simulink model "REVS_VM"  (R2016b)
settings: Solver=ode3  StartTime=REVS.sim_start_time_secs  StopTime=Inf  FixedStep=REVS.sim_step_time_secs  MaxStep=REVS.sim_step_time_secs  EnableMultiTasking=on
StopFcn:
  | postproc_datalog;
  | postproc_audit;
  | postproc_result;
model workspace (MATLAB code in the model file):
  other statements: REVS_setup_variants
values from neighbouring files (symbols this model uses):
  accessory = class_accessory_data    [class_test_data.m]
  battery = class_battery_data    [class_accessory_data.m]    (also in class_REVS_electric.m = class_REVS_battery)
  brake = struct(	'max_torque_Nm',[], 						'proportion_norm',1.0, 						'inertia_kgm2',0.0)    [class_REVS_drive_axle.m]
  engine = class_engine_data    [class_test_data.m]
  final_drive = struct(	'gear_ratio',[], 								'efficiency_norm',[], 								'inertia_kgm2',[] )    [class_REVS_drive_axle.m]
  gear = class_REVS_gearbox    [class_REVS_AT_transmission.m]
  tire = struct(	'radius_m',[], 						'rolling_resistance_coefficient',0, 						'vehicle_weight_norm',1.0,  						'wheel_slip_torque_Nm',[],  						'inertia_kgm2',0.0)    [class_REVS_drive_axle.m]
  torque_converter = class_REVS_torque_converter    [class_REVS_AT_transmission.m]
  transmission = class_transmission_data    [class_test_data.m]
  vehicle = class_vehicle_data    [class_test_data.m]
undefined symbols (not defined in the file or in its folder): alternator, ambient, controls, convert, DelayTimeSecs, drive_cycle, driver, electric, gear_strategy, InitialCondition, InitialValue, LoadSource, LookupStructure, MultiplyPosInputs, Normalize, NumPhases, REVS, SpeedSource, starter, tableshift, UpperSaturationLimit, Value, VerboseLevel, VerboseSignal
libraries: simulink x153
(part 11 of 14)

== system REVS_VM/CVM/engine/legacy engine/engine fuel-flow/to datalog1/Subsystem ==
  In1 : Inport
  Enable : EnablePort
  To Workspace : ToWorkspace  VariableName=datalog__engine__tipin_penalty_gps  SampleTime=-1
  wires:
  In1/1 -> To Workspace/1

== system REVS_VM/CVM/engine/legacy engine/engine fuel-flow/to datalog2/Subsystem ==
  In1 : Inport
  Enable : EnablePort
  To Workspace : ToWorkspace  VariableName=datalog__engine__base_fuel_rate_gps  SampleTime=-1
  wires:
  In1/1 -> To Workspace/1

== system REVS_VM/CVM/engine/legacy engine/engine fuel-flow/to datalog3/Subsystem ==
  In1 : Inport
  Enable : EnablePort
  To Workspace : ToWorkspace  VariableName=datalog__engine__twoD_eng_trq_Nm  SampleTime=-1
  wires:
  In1/1 -> To Workspace/1

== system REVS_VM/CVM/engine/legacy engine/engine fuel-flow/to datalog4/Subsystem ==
  In1 : Inport
  Enable : EnablePort
  To Workspace : ToWorkspace  VariableName=datalog__engine__twoD_eng_spd_radps  SampleTime=-1
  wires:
  In1/1 -> To Workspace/1

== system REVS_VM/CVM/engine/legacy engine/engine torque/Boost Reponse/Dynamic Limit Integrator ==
  upper : Inport
  In : Inport  Port=2
  rst : Inport  Port=3
  Xo : Inport  Port=4
  lower : Inport  Port=5
  Integrator : Integrator  ExternalReset=level  InitialConditionSource=external  ShowStatePort=on
  Logical Operator : Logic  Operator=OR  Inputs=3  AllPortsSameDT=off  OutDataTypeStr=boolean
  lower limit : MinMax  Function=max  Inputs=2  ZeroCross=off
  lower saturation : RelationalOperator  Operator=<  OutDataTypeStr=boolean
  manual reset : Switch  Criteria=u2 ~= 0
  upper limit : MinMax  Inputs=2
  upper saturation : RelationalOperator  Operator=>  OutDataTypeStr=boolean
  Out : Outport
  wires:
  manual reset/1 -> lower limit/1
  upper/1 -> upper limit/1, upper saturation/2
  upper limit/1 -> Integrator/3
  lower/1 -> lower saturation/2, lower limit/2
  In/1 -> Integrator/1
  Logical Operator/1 -> Integrator/2
  lower saturation/1 -> Logical Operator/2
  upper saturation/1 -> Logical Operator/1
  rst/1 -> Logical Operator/3, manual reset/2
  Xo/1 -> manual reset/1
  lower limit/1 -> upper limit/2
  Integrator/1 -> Out/1
  Integrator/State -> upper saturation/1, lower saturation/1, manual reset/3

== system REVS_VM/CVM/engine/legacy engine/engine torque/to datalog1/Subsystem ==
  In1 : Inport
  Enable : EnablePort
  To Workspace : ToWorkspace  VariableName=datalog__engine__load_Nm  SampleTime=-1
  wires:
  In1/1 -> To Workspace/1

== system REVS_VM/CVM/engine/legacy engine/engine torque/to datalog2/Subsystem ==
  In1 : Inport
  Enable : EnablePort
  To Workspace : ToWorkspace  VariableName=datalog__engine__load_norm  SampleTime=-1
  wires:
  In1/1 -> To Workspace/1

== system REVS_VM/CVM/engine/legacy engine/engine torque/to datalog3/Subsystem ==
  In1 : Inport
  Enable : EnablePort
  To Workspace : ToWorkspace  VariableName=datalog__engine__available_torque_Nm  SampleTime=-1
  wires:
  In1/1 -> To Workspace/1

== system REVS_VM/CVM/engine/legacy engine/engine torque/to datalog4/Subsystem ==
  In1 : Inport
  Enable : EnablePort
  To Workspace : ToWorkspace  VariableName=datalog__engine__fueling_torque_Nm  SampleTime=-1
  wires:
  In1/1 -> To Workspace/1

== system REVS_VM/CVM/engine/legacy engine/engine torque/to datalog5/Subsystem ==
  In1 : Inport
  Enable : EnablePort
  To Workspace : ToWorkspace  VariableName=datalog__engine__slow_target_torque_Nm  SampleTime=-1
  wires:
  In1/1 -> To Workspace/1

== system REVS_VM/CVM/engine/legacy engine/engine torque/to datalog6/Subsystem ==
  In1 : Inport
  Enable : EnablePort
  To Workspace : ToWorkspace  VariableName=datalog__engine__fast_target_torque_Nm  SampleTime=-1
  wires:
  In1/1 -> To Workspace/1

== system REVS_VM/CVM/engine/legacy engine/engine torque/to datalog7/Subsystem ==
  In1 : Inport
  Enable : EnablePort
  To Workspace : ToWorkspace  VariableName=datalog__engine__naturally_aspirated_torque_Nm  SampleTime=-1
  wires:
  In1/1 -> To Workspace/1

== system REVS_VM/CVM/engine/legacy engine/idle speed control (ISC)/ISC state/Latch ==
  On : Inport  PortDimensions=1
  Off : Inport  Port=2  PortDimensions=1
  Combinatorial  Logic : CombinatorialLogic  TruthTable=[0;1;0;0;1;1;(tb==2);(tb>=2)]
  Memory2 : Memory  X0=InitialCondition
  Mux : Mux  Inputs=3
  State : Outport  PortDimensions=1
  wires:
  Off/1 -> Mux/2
  On/1 -> Mux/1
  Memory2/1 -> Mux/3
  Mux/1 -> Combinatorial  Logic/1
  Combinatorial  Logic/1 -> State/1, Memory2/1

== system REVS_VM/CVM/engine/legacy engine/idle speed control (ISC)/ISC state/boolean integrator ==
  bool : Inport
  Constant : Constant  Value=Normalize
  Data Type Conversion2 : DataTypeConversion  OutDataTypeStr=double
  Integrator1 : Integrator  ExternalReset=falling  LimitOutput=on  UpperSaturationLimit=UpperSaturationLimit  LowerSaturationLimit=0
  Switch : Switch  Criteria=u2 > Threshold
  normalize : Gain  Gain=1/UpperSaturationLimit
  out : Outport
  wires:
  Switch/1 -> out/1
  normalize/1 -> Switch/1
  Integrator1/1 -> Switch/3, normalize/1
  Constant/1 -> Switch/2
  bool/1 -> Data Type Conversion2/1
  Data Type Conversion2/1 -> Integrator1/1, Integrator1/2

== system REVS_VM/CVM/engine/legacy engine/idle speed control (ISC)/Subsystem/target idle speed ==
  bus : Inport
  Bus Selector : BusSelector  OutputSignals=gb.gb_cmd_gear,gb_spd_in_radps,ctrl.gb_line_press_bar
  Lookup : Lookup_n-D  NumberOfTableDimensions=10  BreakpointsForDimension1=LookupStructure.axis_1.breakpoints  BreakpointsForDimension2=LookupStructure.axis_2.breakpoints  BreakpointsForDimension3=LookupStructure.axis_3.breakpoints  BreakpointsForDimension4=LookupStructure.axis_4.breakpoints  BreakpointsForDimension5=LookupStructure.axis_5.breakpoints  BreakpointsForDimension6=LookupStructure.axis_6.breakpoints  BreakpointsForDimension7=LookupStructure.axis_7.breakpoints  BreakpointsForDimension8=LookupStructure.axis_8.breakpoints  BreakpointsForDimension9=LookupStructure.axis_9.breakpoints  BreakpointsForDimension10=LookupStructure.axis_10.breakpoints  IndexSearchMethod=Linear search  BeginIndexSearchUsingPreviousIndexResult=on  Table=LookupStructure.table  InternalRulePriority=Speed  RndMeth=Simplest  SupportTunableTableSize=on  MaximumIndicesForEachDimension=LookupStructure.table_size
  out : Outport
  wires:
  bus/1 -> Bus Selector/1
  Lookup/1 -> out/1

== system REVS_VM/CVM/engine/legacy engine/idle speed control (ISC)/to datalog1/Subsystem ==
  In1 : Inport
  Enable : EnablePort
  To Workspace : ToWorkspace  VariableName=datalog__engine__ISC_torque_Nm  SampleTime=-1
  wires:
  In1/1 -> To Workspace/1

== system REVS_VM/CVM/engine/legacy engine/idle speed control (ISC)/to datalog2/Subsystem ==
  In1 : Inport
  Enable : EnablePort
  To Workspace : ToWorkspace  VariableName=datalog__engine__ISC_Ki_torque_Nm  SampleTime=-1
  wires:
  In1/1 -> To Workspace/1

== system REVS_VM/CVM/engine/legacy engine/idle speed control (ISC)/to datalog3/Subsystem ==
  In1 : Inport
  Enable : EnablePort
  To Workspace : ToWorkspace  VariableName=datalog__engine__ISC_Kp_torque_Nm  SampleTime=-1
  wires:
  In1/1 -> To Workspace/1

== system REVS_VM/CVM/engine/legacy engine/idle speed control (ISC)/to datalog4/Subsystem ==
  In1 : Inport
  Enable : EnablePort
  To Workspace : ToWorkspace  VariableName=datalog__engine__ISC_Ialpha_Nm  SampleTime=-1
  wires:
  In1/1 -> To Workspace/1

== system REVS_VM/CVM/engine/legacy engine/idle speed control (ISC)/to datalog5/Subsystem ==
  In1 : Inport
  Enable : EnablePort
  To Workspace : ToWorkspace  VariableName=datalog__engine__ISC_target_speed_radps  SampleTime=-1
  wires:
  In1/1 -> To Workspace/1

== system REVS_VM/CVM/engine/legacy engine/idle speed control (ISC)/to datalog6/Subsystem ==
  In1 : Inport
  Enable : EnablePort
  To Workspace : ToWorkspace  VariableName=datalog__engine__ISC_state  SampleTime=-1
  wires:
  In1/1 -> To Workspace/1

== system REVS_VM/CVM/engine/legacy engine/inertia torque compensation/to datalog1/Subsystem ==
  In1 : Inport
  Enable : EnablePort
  To Workspace : ToWorkspace  VariableName=datalog__engine__inertia_comp_torque_Nm  SampleTime=-1
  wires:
  In1/1 -> To Workspace/1

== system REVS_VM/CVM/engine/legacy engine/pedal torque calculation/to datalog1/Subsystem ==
  In1 : Inport
  Enable : EnablePort
  To Workspace : ToWorkspace  VariableName=datalog__engine__accel_pedal_torque_Nm  SampleTime=-1
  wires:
  In1/1 -> To Workspace/1

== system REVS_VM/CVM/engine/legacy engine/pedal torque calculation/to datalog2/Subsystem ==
  In1 : Inport
  Enable : EnablePort
  To Workspace : ToWorkspace  VariableName=datalog__engine__accel_pedal_power_W  SampleTime=-1
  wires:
  In1/1 -> To Workspace/1

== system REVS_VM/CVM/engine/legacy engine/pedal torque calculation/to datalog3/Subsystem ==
  In1 : Inport
  Enable : EnablePort
  To Workspace : ToWorkspace  VariableName=datalog__engine__current_available_power_W  SampleTime=-1
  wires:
  In1/1 -> To Workspace/1

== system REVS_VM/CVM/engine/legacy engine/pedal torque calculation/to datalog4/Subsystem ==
  In1 : Inport
  Enable : EnablePort
  To Workspace : ToWorkspace  VariableName=datalog__engine__current_available_torque_Nm  SampleTime=-1
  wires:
  In1/1 -> To Workspace/1

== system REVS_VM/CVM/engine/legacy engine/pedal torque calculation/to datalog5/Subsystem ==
  In1 : Inport
  Enable : EnablePort
  To Workspace : ToWorkspace  VariableName=datalog__engine__current_min_torque_Nm  SampleTime=-1
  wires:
  In1/1 -> To Workspace/1

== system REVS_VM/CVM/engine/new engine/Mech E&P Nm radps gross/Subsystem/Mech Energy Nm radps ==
  trq_Nm : Inport
  spd_radps : Inport  Port=2
  Gain : Gain  Gain=-1
  Integrator : Integrator  ZeroCross=off
  Integrator1 : Integrator  ZeroCross=off
  Integrator2 : Integrator  ZeroCross=off
  Mux : Mux  Inputs=2
  Neg : Fcn  Expr=u(1)*(u(1) <= 0)
  Pos : Fcn  Expr=u(1)*(u(1) >= 0)
  calc_Power_kW : Fcn  Expr=u(1)*u(2)/1000
  "total_kJ " : Outport
  "pos_kJ " : Outport  Port=2
  neg_kJ : Outport  Port=3
  pwr_kW : Outport  Port=4
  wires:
  calc_Power_kW/1 -> Pos/1, Neg/1, pwr_kW/1, Integrator/1
  Gain/1 -> neg_kJ/1
  Integrator1/1 -> "pos_kJ "/1
  Integrator2/1 -> Gain/1
  Neg/1 -> Integrator2/1
  Pos/1 -> Integrator1/1
  spd_radps/1 -> Mux/2
  trq_Nm/1 -> Mux/1
  Mux/1 -> calc_Power_kW/1
  Integrator/1 -> "total_kJ "/1

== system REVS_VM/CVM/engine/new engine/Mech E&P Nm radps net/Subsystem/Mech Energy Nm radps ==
  trq_Nm : Inport
  spd_radps : Inport  Port=2
  Gain : Gain  Gain=-1
  Integrator : Integrator  ZeroCross=off
  Integrator1 : Integrator  ZeroCross=off
  Integrator2 : Integrator  ZeroCross=off
  Mux : Mux  Inputs=2
  Neg : Fcn  Expr=u(1)*(u(1) <= 0)
  Pos : Fcn  Expr=u(1)*(u(1) >= 0)
  calc_Power_kW : Fcn  Expr=u(1)*u(2)/1000
  "total_kJ " : Outport
  "pos_kJ " : Outport  Port=2
  neg_kJ : Outport  Port=3
  pwr_kW : Outport  Port=4
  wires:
  calc_Power_kW/1 -> Pos/1, Neg/1, pwr_kW/1, Integrator/1
  Gain/1 -> neg_kJ/1
  Integrator1/1 -> "pos_kJ "/1
  Integrator2/1 -> Gain/1
  Neg/1 -> Integrator2/1
  Pos/1 -> Integrator1/1
  spd_radps/1 -> Mux/2
  trq_Nm/1 -> Mux/1
  Mux/1 -> calc_Power_kW/1
  Integrator/1 -> "total_kJ "/1

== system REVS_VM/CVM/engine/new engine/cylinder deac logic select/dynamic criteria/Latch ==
  On : Inport  PortDimensions=1
  Off : Inport  Port=2  PortDimensions=1
  Combinatorial  Logic : CombinatorialLogic  TruthTable=[0;1;0;0;1;1;(tb==2);(tb>=2)]
  Memory2 : Memory  X0=InitialCondition
  Mux : Mux  Inputs=3
  State : Outport  PortDimensions=1
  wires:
  Off/1 -> Mux/2
  On/1 -> Mux/1
  Memory2/1 -> Mux/3
  Mux/1 -> Combinatorial  Logic/1
  Combinatorial  Logic/1 -> State/1, Memory2/1

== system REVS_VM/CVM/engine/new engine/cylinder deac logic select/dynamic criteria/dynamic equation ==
  bus : Inport
  Bus Creator : BusCreator  Inputs=10
  Bus Creator1 : BusCreator  Inputs=2
  Bus Selector : BusSelector  OutputSignals=var_sigs.var_sig1  OutputAsBus=on
  Data Type Conversion : DataTypeConversion  OutDataTypeStr=double
  Display : Display
  Fcn : Fcn
  Variable {1..10} (10 alike) : Constant  Value=nan
  out : Outport
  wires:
  Data Type Conversion/1 -> Fcn/1
  Bus Selector/1 -> Data Type Conversion/1, Display/1
  Bus Creator1/1 -> Bus Selector/1
  Fcn/1 -> out/1
  bus/1 -> Bus Creator1/1  "system_bus"
  Bus Creator/1 -> Bus Creator1/2  "var_sigs"
  Variable 1/1 -> Bus Creator/1  "var_sig1"
  Variable 2/1 -> Bus Creator/2  "var_sig2"
  Variable 3/1 -> Bus Creator/3  "var_sig3"
  Variable 4/1 -> Bus Creator/4  "var_sig4"
  Variable 5/1 -> Bus Creator/5  "var_sig5"
  Variable 6/1 -> Bus Creator/6  "var_sig6"
  Variable 7/1 -> Bus Creator/7  "var_sig7"
  Variable 8/1 -> Bus Creator/8  "var_sig8"
  Variable 9/1 -> Bus Creator/9  "var_sig9"
  Variable 10/1 -> Bus Creator/10  "var_sig10"

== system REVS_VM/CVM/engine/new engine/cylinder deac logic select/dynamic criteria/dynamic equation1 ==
  bus : Inport
  Bus Creator : BusCreator  Inputs=10
  Bus Creator1 : BusCreator  Inputs=2
  Bus Selector : BusSelector  OutputSignals=var_sigs.var_sig1  OutputAsBus=on
  Data Type Conversion : DataTypeConversion  OutDataTypeStr=double
  Display : Display
  Fcn : Fcn
  Variable {1..10} (10 alike) : Constant  Value=nan
  out : Outport
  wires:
  Data Type Conversion/1 -> Fcn/1
  Bus Selector/1 -> Data Type Conversion/1, Display/1
  Bus Creator1/1 -> Bus Selector/1
  Fcn/1 -> out/1
  bus/1 -> Bus Creator1/1  "system_bus"
  Bus Creator/1 -> Bus Creator1/2  "var_sigs"
  Variable 1/1 -> Bus Creator/1  "var_sig1"
  Variable 2/1 -> Bus Creator/2  "var_sig2"
  Variable 3/1 -> Bus Creator/3  "var_sig3"
  Variable 4/1 -> Bus Creator/4  "var_sig4"
  Variable 5/1 -> Bus Creator/5  "var_sig5"
  Variable 6/1 -> Bus Creator/6  "var_sig6"
  Variable 7/1 -> Bus Creator/7  "var_sig7"
  Variable 8/1 -> Bus Creator/8  "var_sig8"
  Variable 9/1 -> Bus Creator/9  "var_sig9"
  Variable 10/1 -> Bus Creator/10  "var_sig10"

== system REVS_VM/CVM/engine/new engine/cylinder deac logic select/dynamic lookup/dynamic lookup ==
  bus : Inport
  Bus Selector : BusSelector  OutputSignals=gb.gb_cmd_gear,gb_spd_in_radps,ctrl.gb_line_press_bar
  Lookup : Lookup_n-D  NumberOfTableDimensions=10  BreakpointsForDimension1=LookupStructure.axis_1.breakpoints  BreakpointsForDimension2=LookupStructure.axis_2.breakpoints  BreakpointsForDimension3=LookupStructure.axis_3.breakpoints  BreakpointsForDimension4=LookupStructure.axis_4.breakpoints  BreakpointsForDimension5=LookupStructure.axis_5.breakpoints  BreakpointsForDimension6=LookupStructure.axis_6.breakpoints  BreakpointsForDimension7=LookupStructure.axis_7.breakpoints  BreakpointsForDimension8=LookupStructure.axis_8.breakpoints  BreakpointsForDimension9=LookupStructure.axis_9.breakpoints  BreakpointsForDimension10=LookupStructure.axis_10.breakpoints  IndexSearchMethod=Linear search  BeginIndexSearchUsingPreviousIndexResult=on  Table=LookupStructure.table  DiagnosticForOutOfRangeInput=Warning  InternalRulePriority=Speed  RndMeth=Simplest  SupportTunableTableSize=on  MaximumIndicesForEachDimension=LookupStructure.table_size
  out : Outport
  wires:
  bus/1 -> Bus Selector/1
  Lookup/1 -> out/1

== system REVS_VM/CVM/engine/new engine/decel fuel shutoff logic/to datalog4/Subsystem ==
  In1 : Inport
  Enable : EnablePort
  To Workspace : ToWorkspace  VariableName=datalog__engine__dfco_active_bool  SampleTime=-1
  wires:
  In1/1 -> To Workspace/1

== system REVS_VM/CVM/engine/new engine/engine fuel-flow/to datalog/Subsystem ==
  In1 : Inport
  Enable : EnablePort
  To Workspace : ToWorkspace  VariableName=datalog__engine__transient_correction_gps  SampleTime=-1
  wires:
  In1/1 -> To Workspace/1

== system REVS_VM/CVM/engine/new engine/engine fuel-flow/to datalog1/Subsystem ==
  In1 : Inport
  Enable : EnablePort
  To Workspace : ToWorkspace  VariableName=datalog__engine__dfco_refuel_penalty_gps  SampleTime=-1
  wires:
  In1/1 -> To Workspace/1

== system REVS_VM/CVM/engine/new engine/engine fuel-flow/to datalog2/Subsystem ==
  In1 : Inport
  Enable : EnablePort
  To Workspace : ToWorkspace  VariableName=datalog__engine__base_fuel_rate_gps  SampleTime=-1
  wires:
  In1/1 -> To Workspace/1

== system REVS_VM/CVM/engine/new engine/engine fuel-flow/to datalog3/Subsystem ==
  In1 : Inport
  Enable : EnablePort
  To Workspace : ToWorkspace  VariableName=datalog__engine__transient_correction_g  SampleTime=-1
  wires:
  In1/1 -> To Workspace/1

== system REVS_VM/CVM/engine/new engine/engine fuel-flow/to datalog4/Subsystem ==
  In1 : Inport
  Enable : EnablePort
  To Workspace : ToWorkspace  VariableName=datalog__engine__dfco_refuel_penalty_g  SampleTime=-1
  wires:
  In1/1 -> To Workspace/1

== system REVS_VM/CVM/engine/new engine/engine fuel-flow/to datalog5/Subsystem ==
  In1 : Inport
  Enable : EnablePort
  To Workspace : ToWorkspace  VariableName=datalog__engine__base_fuel_g  SampleTime=-1
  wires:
  In1/1 -> To Workspace/1

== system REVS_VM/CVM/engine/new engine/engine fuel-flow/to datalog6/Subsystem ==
  In1 : Inport
  Enable : EnablePort
  To Workspace : ToWorkspace  VariableName=datalog__engine__dfco_refuel_timer_s  SampleTime=-1
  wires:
  In1/1 -> To Workspace/1

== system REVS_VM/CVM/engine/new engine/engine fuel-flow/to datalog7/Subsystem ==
  In1 : Inport
  Enable : EnablePort
  To Workspace : ToWorkspace  VariableName=datalog__engine__deac_transition_penalty_gps  SampleTime=-1
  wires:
  In1/1 -> To Workspace/1

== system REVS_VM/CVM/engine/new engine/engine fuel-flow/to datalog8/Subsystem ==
  In1 : Inport
  Enable : EnablePort
  To Workspace : ToWorkspace  VariableName=datalog__engine__deac_transition_penalty_g  SampleTime=-1
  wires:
  In1/1 -> To Workspace/1

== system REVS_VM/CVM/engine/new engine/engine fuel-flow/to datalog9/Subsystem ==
  In1 : Inport
  Enable : EnablePort
  To Workspace : ToWorkspace  VariableName=datalog__engine__deac_off_timer_s  SampleTime=-1
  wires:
  In1/1 -> To Workspace/1

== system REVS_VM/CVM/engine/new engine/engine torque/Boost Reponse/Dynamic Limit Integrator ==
  upper : Inport
  In : Inport  Port=2
  rst : Inport  Port=3
  Xo : Inport  Port=4
  lower : Inport  Port=5
  Integrator : Integrator  ExternalReset=level  InitialConditionSource=external  ShowStatePort=on
  Logical Operator : Logic  Operator=OR  Inputs=3  AllPortsSameDT=off  OutDataTypeStr=boolean
  lower limit : MinMax  Function=max  Inputs=2  ZeroCross=off
  lower saturation : RelationalOperator  Operator=<  OutDataTypeStr=boolean
  manual reset : Switch  Criteria=u2 ~= 0
  upper limit : MinMax  Inputs=2
  upper saturation : RelationalOperator  Operator=>  OutDataTypeStr=boolean
  Out : Outport
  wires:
  manual reset/1 -> lower limit/1
  upper/1 -> upper limit/1, upper saturation/2
  upper limit/1 -> Integrator/3
  lower/1 -> lower saturation/2, lower limit/2
  In/1 -> Integrator/1
  Logical Operator/1 -> Integrator/2
  lower saturation/1 -> Logical Operator/2
  upper saturation/1 -> Logical Operator/1
  rst/1 -> Logical Operator/3, manual reset/2
  Xo/1 -> manual reset/1
  lower limit/1 -> upper limit/2
  Integrator/1 -> Out/1
  Integrator/State -> upper saturation/1, lower saturation/1, manual reset/3

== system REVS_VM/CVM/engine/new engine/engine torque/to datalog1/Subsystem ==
  In1 : Inport
  Enable : EnablePort
  To Workspace : ToWorkspace  VariableName=datalog__engine__load_Nm  SampleTime=-1
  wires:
  In1/1 -> To Workspace/1

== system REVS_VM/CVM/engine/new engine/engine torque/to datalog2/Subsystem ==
  In1 : Inport
  Enable : EnablePort
  To Workspace : ToWorkspace  VariableName=datalog__engine__load_norm  SampleTime=-1
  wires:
  In1/1 -> To Workspace/1

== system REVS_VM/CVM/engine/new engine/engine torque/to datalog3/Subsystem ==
  In1 : Inport
  Enable : EnablePort
  To Workspace : ToWorkspace  VariableName=datalog__engine__available_torque_Nm  SampleTime=-1
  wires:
  In1/1 -> To Workspace/1

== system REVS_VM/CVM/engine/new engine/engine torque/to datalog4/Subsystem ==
  In1 : Inport
  Enable : EnablePort
  To Workspace : ToWorkspace  VariableName=datalog__engine__fueling_torque_Nm  SampleTime=-1
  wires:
  In1/1 -> To Workspace/1

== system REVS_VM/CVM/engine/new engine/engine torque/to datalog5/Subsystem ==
  In1 : Inport
  Enable : EnablePort
  To Workspace : ToWorkspace  VariableName=datalog__engine__slow_target_torque_Nm  SampleTime=-1
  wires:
  In1/1 -> To Workspace/1

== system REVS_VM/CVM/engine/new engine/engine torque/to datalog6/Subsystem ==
  In1 : Inport
  Enable : EnablePort
  To Workspace : ToWorkspace  VariableName=datalog__engine__fast_target_torque_Nm  SampleTime=-1
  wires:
  In1/1 -> To Workspace/1

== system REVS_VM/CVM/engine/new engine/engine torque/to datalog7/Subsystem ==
  In1 : Inport
  Enable : EnablePort
  To Workspace : ToWorkspace  VariableName=datalog__engine__naturally_aspirated_torque_Nm  SampleTime=-1
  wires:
  In1/1 -> To Workspace/1

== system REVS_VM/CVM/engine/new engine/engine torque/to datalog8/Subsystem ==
  In1 : Inport
  Enable : EnablePort
  To Workspace : ToWorkspace  VariableName=datalog__engine__available_power_W  SampleTime=-1
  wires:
  In1/1 -> To Workspace/1

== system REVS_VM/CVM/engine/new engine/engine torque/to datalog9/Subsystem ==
  In1 : Inport
  Enable : EnablePort
  To Workspace : ToWorkspace  VariableName=datalog__engine__throttle_pos_norm  SampleTime=-1
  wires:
  In1/1 -> To Workspace/1

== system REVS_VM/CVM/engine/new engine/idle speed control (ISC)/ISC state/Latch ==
  On : Inport  PortDimensions=1
  Off : Inport  Port=2  PortDimensions=1
  Combinatorial  Logic : CombinatorialLogic  TruthTable=[0;1;0;0;1;1;(tb==2);(tb>=2)]
  Memory2 : Memory  X0=InitialCondition
  Mux : Mux  Inputs=3
  State : Outport  PortDimensions=1
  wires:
  Off/1 -> Mux/2
  On/1 -> Mux/1
  Memory2/1 -> Mux/3
  Mux/1 -> Combinatorial  Logic/1
  Combinatorial  Logic/1 -> State/1, Memory2/1

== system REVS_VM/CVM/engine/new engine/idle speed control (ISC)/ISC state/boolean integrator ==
  bool : Inport
  Constant : Constant  Value=Normalize
  Data Type Conversion2 : DataTypeConversion  OutDataTypeStr=double
  Integrator1 : Integrator  ExternalReset=falling  LimitOutput=on  UpperSaturationLimit=UpperSaturationLimit  LowerSaturationLimit=0
  Switch : Switch  Criteria=u2 > Threshold
  normalize : Gain  Gain=1/UpperSaturationLimit
  out : Outport
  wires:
  Switch/1 -> out/1
  normalize/1 -> Switch/1
  Integrator1/1 -> Switch/3, normalize/1
  Constant/1 -> Switch/2
  bool/1 -> Data Type Conversion2/1
  Data Type Conversion2/1 -> Integrator1/1, Integrator1/2

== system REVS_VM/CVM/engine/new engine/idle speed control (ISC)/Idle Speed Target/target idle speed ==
  bus : Inport
  Bus Selector : BusSelector  OutputSignals=gb.gb_cmd_gear,gb_spd_in_radps,ctrl.gb_line_press_bar
  Lookup : Lookup_n-D  NumberOfTableDimensions=10  BreakpointsForDimension1=LookupStructure.axis_1.breakpoints  BreakpointsForDimension2=LookupStructure.axis_2.breakpoints  BreakpointsForDimension3=LookupStructure.axis_3.breakpoints  BreakpointsForDimension4=LookupStructure.axis_4.breakpoints  BreakpointsForDimension5=LookupStructure.axis_5.breakpoints  BreakpointsForDimension6=LookupStructure.axis_6.breakpoints  BreakpointsForDimension7=LookupStructure.axis_7.breakpoints  BreakpointsForDimension8=LookupStructure.axis_8.breakpoints  BreakpointsForDimension9=LookupStructure.axis_9.breakpoints  BreakpointsForDimension10=LookupStructure.axis_10.breakpoints  IndexSearchMethod=Linear search  BeginIndexSearchUsingPreviousIndexResult=on  Table=LookupStructure.table  InternalRulePriority=Speed  RndMeth=Simplest  SupportTunableTableSize=on  MaximumIndicesForEachDimension=LookupStructure.table_size
  out : Outport
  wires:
  bus/1 -> Bus Selector/1
  Lookup/1 -> out/1

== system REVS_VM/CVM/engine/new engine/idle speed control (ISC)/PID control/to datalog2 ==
  Var : Inport
  Constant : Constant  Value=VerboseSignal
  Constant1 : Constant  Value=VerboseLevel
  Relational Operator : RelationalOperator  OutDataTypeStr=boolean  ZeroCross=off
  Subsystem : Subsystem
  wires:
  Constant1/1 -> Relational Operator/2
  Constant/1 -> Relational Operator/1
  Relational Operator/1 -> Subsystem/Enable
  Var/1 -> Subsystem/1(In1)

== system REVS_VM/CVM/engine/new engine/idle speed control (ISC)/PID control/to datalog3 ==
  Var : Inport
  Constant : Constant  Value=VerboseSignal
  Constant1 : Constant  Value=VerboseLevel
  Relational Operator : RelationalOperator  OutDataTypeStr=boolean  ZeroCross=off
  Subsystem : Subsystem
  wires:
  Constant1/1 -> Relational Operator/2
  Constant/1 -> Relational Operator/1
  Relational Operator/1 -> Subsystem/Enable
  Var/1 -> Subsystem/1(In1)

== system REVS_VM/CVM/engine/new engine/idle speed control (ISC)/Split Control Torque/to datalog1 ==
  Var : Inport
  Constant : Constant  Value=VerboseSignal
  Constant1 : Constant  Value=VerboseLevel
  Relational Operator : RelationalOperator  OutDataTypeStr=boolean  ZeroCross=off
  Subsystem : Subsystem
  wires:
  Constant1/1 -> Relational Operator/2
  Constant/1 -> Relational Operator/1
  Relational Operator/1 -> Subsystem/Enable
  Var/1 -> Subsystem/1(In1)

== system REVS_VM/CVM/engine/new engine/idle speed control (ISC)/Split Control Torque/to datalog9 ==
  Var : Inport
  Constant : Constant  Value=VerboseSignal
  Constant1 : Constant  Value=VerboseLevel
  Relational Operator : RelationalOperator  OutDataTypeStr=boolean  ZeroCross=off
  Subsystem : Subsystem
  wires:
  Constant1/1 -> Relational Operator/2
  Constant/1 -> Relational Operator/1
  Relational Operator/1 -> Subsystem/Enable
  Var/1 -> Subsystem/1(In1)

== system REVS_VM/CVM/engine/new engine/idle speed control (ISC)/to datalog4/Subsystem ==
  In1 : Inport
  Enable : EnablePort
  To Workspace : ToWorkspace  VariableName=datalog__engine__ISC_Ialpha_Nm  SampleTime=-1
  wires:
  In1/1 -> To Workspace/1

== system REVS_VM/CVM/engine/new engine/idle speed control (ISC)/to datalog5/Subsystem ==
  In1 : Inport
  Enable : EnablePort
  To Workspace : ToWorkspace  VariableName=datalog__engine__ISC_target_speed_radps  SampleTime=-1
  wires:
  In1/1 -> To Workspace/1

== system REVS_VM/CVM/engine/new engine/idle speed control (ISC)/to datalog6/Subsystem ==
  In1 : Inport
  Enable : EnablePort
  To Workspace : ToWorkspace  VariableName=datalog__engine__ISC_state  SampleTime=-1
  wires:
  In1/1 -> To Workspace/1

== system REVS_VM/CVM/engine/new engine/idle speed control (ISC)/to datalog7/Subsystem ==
  In1 : Inport
  Enable : EnablePort
  To Workspace : ToWorkspace  VariableName=datalog__engine__ISC_slow_torque_Nm  SampleTime=-1
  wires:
  In1/1 -> To Workspace/1

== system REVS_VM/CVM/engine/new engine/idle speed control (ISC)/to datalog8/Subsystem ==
  In1 : Inport
  Enable : EnablePort
  To Workspace : ToWorkspace  VariableName=datalog__engine__ISC_fast_torque_Nm  SampleTime=-1
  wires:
  In1/1 -> To Workspace/1

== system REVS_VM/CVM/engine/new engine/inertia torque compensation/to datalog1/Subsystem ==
  In1 : Inport
  Enable : EnablePort
  To Workspace : ToWorkspace  VariableName=datalog__engine__inertia_comp_torque_Nm  SampleTime=-1
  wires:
  In1/1 -> To Workspace/1

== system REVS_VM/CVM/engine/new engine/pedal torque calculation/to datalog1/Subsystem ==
  In1 : Inport
  Enable : EnablePort
  To Workspace : ToWorkspace  VariableName=datalog__engine__accel_pedal_torque_Nm  SampleTime=-1
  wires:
  In1/1 -> To Workspace/1

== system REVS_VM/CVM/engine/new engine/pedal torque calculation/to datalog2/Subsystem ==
  In1 : Inport
  Enable : EnablePort
  To Workspace : ToWorkspace  VariableName=datalog__engine__accel_pedal_power_W  SampleTime=-1
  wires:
  In1/1 -> To Workspace/1

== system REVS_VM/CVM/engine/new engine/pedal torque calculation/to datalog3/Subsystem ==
  In1 : Inport
  Enable : EnablePort
  To Workspace : ToWorkspace  VariableName=datalog__engine__accel_pedal_gross_torque_Nm  SampleTime=-1
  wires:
  In1/1 -> To Workspace/1

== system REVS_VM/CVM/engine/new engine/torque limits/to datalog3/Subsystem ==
  In1 : Inport
  Enable : EnablePort
  To Workspace : ToWorkspace  VariableName=datalog__engine__current_available_power_W  SampleTime=-1
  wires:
  In1/1 -> To Workspace/1

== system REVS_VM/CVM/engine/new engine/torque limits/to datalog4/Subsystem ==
  In1 : Inport
  Enable : EnablePort
  To Workspace : ToWorkspace  VariableName=datalog__engine__current_available_torque_Nm  SampleTime=-1
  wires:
  In1/1 -> To Workspace/1

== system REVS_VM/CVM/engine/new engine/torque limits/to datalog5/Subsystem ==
  In1 : Inport
  Enable : EnablePort
  To Workspace : ToWorkspace  VariableName=datalog__engine__current_min_torque_Nm  SampleTime=-1
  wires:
  In1/1 -> To Workspace/1

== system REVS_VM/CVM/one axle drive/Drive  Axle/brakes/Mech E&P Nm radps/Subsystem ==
  " trq_Nm" : Inport
  spd_radps : Inport  Port=2
  iner_kgm2 : Inport  Port=3
  Enable : EnablePort  ZeroCross=off
  KE_to_workspace : ToWorkspace  VariableName=audit__mech__drive_axle1__brake_KE_kJ  SampleTime=-1
  Mech Energy Nm radps : Subsystem  TreatAsAtomicUnit=on
  Mult : Product  Inputs=**
  Square : Math  Operator=square
  energy_to_workspace : ToWorkspace  VariableName=audit__mech__drive_axle1__brake_kJ  SampleTime=-1
  inertia_to_workspace : ToWorkspace  VariableName=audit__mech__drive_axle1__brake_kgm2  SampleTime=-1
  neg_energy_to_workspace : ToWorkspace  VariableName=audit__mech__drive_axle1__brake_neg_kJ  SampleTime=-1
  one half : Gain  Gain=0.5/1000
  pos_energy_to_workspace : ToWorkspace  VariableName=audit__mech__drive_axle1__brake_pos_kJ  SampleTime=-1
  power_to_workspace : ToWorkspace  VariableName=audit__mech__drive_axle1__brake_kW  SampleTime=-1
  speed_to_workspace : ToWorkspace  VariableName=audit__mech__drive_axle1__brake_radps  SampleTime=-1
  torque_to_workspace : ToWorkspace  VariableName=audit__mech__drive_axle1__brake_Nm  SampleTime=-1
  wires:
  Mult/1 -> one half/1
  Square/1 -> Mult/1
  one half/1 -> KE_to_workspace/1
  Mech Energy Nm radps/3(neg_kJ) -> neg_energy_to_workspace/1
  Mech Energy Nm radps/2("pos_kJ ") -> pos_energy_to_workspace/1
  Mech Energy Nm radps/4(pwr_kW) -> power_to_workspace/1
  Mech Energy Nm radps/1("total_kJ ") -> energy_to_workspace/1
  iner_kgm2/1 -> inertia_to_workspace/1, Mult/2
  spd_radps/1 -> Mech Energy Nm radps/2(spd_radps), speed_to_workspace/1, Square/1
  " trq_Nm"/1 -> Mech Energy Nm radps/1(trq_Nm), torque_to_workspace/1

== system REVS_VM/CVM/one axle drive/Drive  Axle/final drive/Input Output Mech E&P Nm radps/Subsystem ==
  trq_in_Nm : Inport
  spd_in_radps : Inport  Port=2
  iner_in_kgm2 : Inport  Port=3
  trq_out_Nm : Inport  Port=4
  spd_out_radps : Inport  Port=5
  iner_out_kgm2 : Inport  Port=6
  Enable : EnablePort  ZeroCross=off
  Input Mech E&P Nm radps : Subsystem
  Loss_KJ_to_workspace : ToWorkspace  VariableName=audit__mech__drive_axle1__final_drive__loss_kJ  SampleTime=-1
  Output Mech E&P Nm radps : Subsystem
  Pos : Saturate  UpperLimit=Inf  LowerLimit=0  ZeroCross=off
  Pos2 : Saturate  UpperLimit=Inf  LowerLimit=0  ZeroCross=off
  Sum : Sum  Inputs=|+-
  Sum1 : Sum  Inputs=-+|
  Sum2 : Sum
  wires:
  Pos2/1 -> Sum2/2
  Pos/1 -> Sum2/1
  trq_in_Nm/1 -> Input Mech E&P Nm radps/1(" trq_Nm")
  spd_in_radps/1 -> Input Mech E&P Nm radps/2(spd_radps)
  trq_out_Nm/1 -> Output Mech E&P Nm radps/1(" trq_Nm")
  spd_out_radps/1 -> Output Mech E&P Nm radps/2(spd_radps)
  iner_in_kgm2/1 -> Input Mech E&P Nm radps/3(iner_kgm2)
  iner_out_kgm2/1 -> Output Mech E&P Nm radps/3(iner_kgm2)
  Input Mech E&P Nm radps/1(pos_kJ) -> Sum/1
  Output Mech E&P Nm radps/1(pos_kJ) -> Sum/2
  Output Mech E&P Nm radps/2(neg_kJ) -> Sum1/2
  Input Mech E&P Nm radps/2(neg_kJ) -> Sum1/1
  Sum/1 -> Pos/1
  Sum1/1 -> Pos2/1
  Sum2/1 -> Loss_KJ_to_workspace/1

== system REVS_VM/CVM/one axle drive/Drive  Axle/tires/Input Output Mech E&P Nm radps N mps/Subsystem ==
  trq_in_Nm : Inport
  spd_in_radps : Inport  Port=2
  iner_in_kgm2 : Inport  Port=3
  frc_out_N : Inport  Port=4
  spd_out_mps : Inport  Port=5
  mass_out_kg : Inport  Port=6
  Enable : EnablePort  ZeroCross=off
  Input Mech E&P Nm radps : Subsystem
  Loss_KJ_to_workspace : ToWorkspace  VariableName=audit__mech__drive_axle1__tire__loss_kJ  SampleTime=-1
  Output Mech E&P N mps : Subsystem
  Pos : Saturate  UpperLimit=Inf  LowerLimit=0  ZeroCross=off
  Pos2 : Saturate  UpperLimit=Inf  LowerLimit=0  ZeroCross=off
  Sum : Sum  Inputs=|+-
  Sum1 : Sum  Inputs=-+|
  Sum2 : Sum
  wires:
  Sum2/1 -> Loss_KJ_to_workspace/1
  Sum1/1 -> Pos2/1
  Sum/1 -> Pos/1
  Input Mech E&P Nm radps/2(neg_kJ) -> Sum1/1
  Output Mech E&P N mps/2(neg_kJ) -> Sum1/2
  Output Mech E&P N mps/1(pos_kJ) -> Sum/2
  Input Mech E&P Nm radps/1(pos_kJ) -> Sum/1
  Pos/1 -> Sum2/1
  Pos2/1 -> Sum2/2
  mass_out_kg/1 -> Output Mech E&P N mps/3(mass_kg)
  iner_in_kgm2/1 -> Input Mech E&P Nm radps/3(iner_kgm2)
  trq_in_Nm/1 -> Input Mech E&P Nm radps/1(" trq_Nm")
  spd_in_radps/1 -> Input Mech E&P Nm radps/2(spd_radps)
  frc_out_N/1 -> Output Mech E&P N mps/1(force_N)
  spd_out_mps/1 -> Output Mech E&P N mps/2(spd_mps)

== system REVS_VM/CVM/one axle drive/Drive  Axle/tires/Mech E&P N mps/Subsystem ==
  force_N : Inport
  spd_mps : Inport  Port=2
  Enable : EnablePort  ZeroCross=off
  Integrator1 : Integrator  LimitOutput=on  UpperSaturationLimit=Inf  LowerSaturationLimit=0  ZeroCross=off
  Mech Energy N mps : Subsystem  TreatAsAtomicUnit=on
  distance_to_workspace : ToWorkspace  VariableName=audit__mech__drive_axle1__tire__rolling_drag_m  SampleTime=-1
  energy_to_workspace : ToWorkspace  VariableName=audit__mech__drive_axle1__tire__rolling_drag_kJ  SampleTime=-1
  force_to_workspace : ToWorkspace  VariableName=audit__mech__drive_axle1__tire__rolling_drag_N  SampleTime=-1
  neg_energy_to_workspace : ToWorkspace  VariableName=audit__mech__drive_axle1__tire__rolling_drag_neg_kJ  SampleTime=-1
  pos_energy_to_workspace : ToWorkspace  VariableName=audit__mech__drive_axle1__tire__rolling_drag_pos_kJ  SampleTime=-1
  power_to_workspace : ToWorkspace  VariableName=audit__mech__drive_axle1__tire__rolling_drag_kW  SampleTime=-1
  speed_to_workspace : ToWorkspace  VariableName=audit__mech__drive_axle1__tire__rolling_drag_mps  SampleTime=-1
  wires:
  Integrator1/1 -> distance_to_workspace/1
  spd_mps/1 -> Mech Energy N mps/2(spd_mps), speed_to_workspace/1, Integrator1/1
  force_N/1 -> Mech Energy N mps/1(force_N), force_to_workspace/1
  Mech Energy N mps/1("total_kJ ") -> energy_to_workspace/1
  Mech Energy N mps/4(pwr_kW) -> power_to_workspace/1
  Mech Energy N mps/2("pos_kJ ") -> pos_energy_to_workspace/1
  Mech Energy N mps/3(neg_kJ) -> neg_energy_to_workspace/1

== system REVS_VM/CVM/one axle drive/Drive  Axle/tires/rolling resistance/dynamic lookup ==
  bus : Inport
  Bus Selector : BusSelector  OutputSignals=gb.gb_cmd_gear,gb_spd_in_radps,ctrl.gb_line_press_bar
  Lookup : Lookup_n-D  NumberOfTableDimensions=10  BreakpointsForDimension1=LookupStructure.axis_1.breakpoints  BreakpointsForDimension2=LookupStructure.axis_2.breakpoints  BreakpointsForDimension3=LookupStructure.axis_3.breakpoints  BreakpointsForDimension4=LookupStructure.axis_4.breakpoints  BreakpointsForDimension5=LookupStructure.axis_5.breakpoints  BreakpointsForDimension6=LookupStructure.axis_6.breakpoints  BreakpointsForDimension7=LookupStructure.axis_7.breakpoints  BreakpointsForDimension8=LookupStructure.axis_8.breakpoints  BreakpointsForDimension9=LookupStructure.axis_9.breakpoints  BreakpointsForDimension10=LookupStructure.axis_10.breakpoints  IndexSearchMethod=Linear search  BeginIndexSearchUsingPreviousIndexResult=on  Table=LookupStructure.table  DiagnosticForOutOfRangeInput=Warning  InternalRulePriority=Speed  RndMeth=Simplest  SupportTunableTableSize=on  MaximumIndicesForEachDimension=LookupStructure.table_size
  out : Outport
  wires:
  bus/1 -> Bus Selector/1
  Lookup/1 -> out/1

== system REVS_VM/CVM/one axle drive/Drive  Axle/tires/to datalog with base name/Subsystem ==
  Var : Inport
  Enable : EnablePort
  To Workspace : ToWorkspace  VariableName=datalog__drive_axle1__tire__slip_pct  SampleTime=-1
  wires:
  Var/1 -> To Workspace/1

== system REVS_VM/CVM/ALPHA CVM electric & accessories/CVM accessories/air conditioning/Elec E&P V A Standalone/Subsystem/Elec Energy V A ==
  volts_V : Inport
  curr_A : Inport  Port=2
  Gain : Gain  Gain=-1
  Integrator : Integrator  ZeroCross=off
  Integrator1 : Integrator  ZeroCross=off
  Integrator2 : Integrator  ZeroCross=off
  Mux : Mux  Inputs=2
  Neg : Fcn  Expr=u(1)*(u(1) <= 0)
  Pos : Fcn  Expr=u(1)*(u(1) >= 0)
  calc_Power_kW : Fcn  Expr=u(1)*u(2)/1000
  "total_kJ " : Outport
  "pos_kJ " : Outport  Port=2
  neg_kJ : Outport  Port=3
  pwr_kW : Outport  Port=4
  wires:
  curr_A/1 -> Mux/2
  volts_V/1 -> Mux/1
  Mux/1 -> calc_Power_kW/1
  Integrator/1 -> "total_kJ "/1
  Pos/1 -> Integrator1/1
  Neg/1 -> Integrator2/1
  Integrator2/1 -> Gain/1
  Integrator1/1 -> "pos_kJ "/1
  Gain/1 -> neg_kJ/1
  calc_Power_kW/1 -> Integrator/1, pwr_kW/1, Neg/1, Pos/1

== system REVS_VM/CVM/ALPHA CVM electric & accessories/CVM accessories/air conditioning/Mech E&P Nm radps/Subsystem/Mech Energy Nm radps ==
  trq_Nm : Inport
  spd_radps : Inport  Port=2
  Gain : Gain  Gain=-1
  Integrator : Integrator  ZeroCross=off
  Integrator1 : Integrator  ZeroCross=off
  Integrator2 : Integrator  ZeroCross=off
  Mux : Mux  Inputs=2
  Neg : Fcn  Expr=u(1)*(u(1) <= 0)
  Pos : Fcn  Expr=u(1)*(u(1) >= 0)
  calc_Power_kW : Fcn  Expr=u(1)*u(2)/1000
  "total_kJ " : Outport
  "pos_kJ " : Outport  Port=2
  neg_kJ : Outport  Port=3
  pwr_kW : Outport  Port=4
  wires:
  calc_Power_kW/1 -> Pos/1, Neg/1, pwr_kW/1, Integrator/1
  Gain/1 -> neg_kJ/1
  Integrator1/1 -> "pos_kJ "/1
  Integrator2/1 -> Gain/1
  Neg/1 -> Integrator2/1
  Pos/1 -> Integrator1/1
  spd_radps/1 -> Mux/2
  trq_Nm/1 -> Mux/1
  Mux/1 -> calc_Power_kW/1
  Integrator/1 -> "total_kJ "/1

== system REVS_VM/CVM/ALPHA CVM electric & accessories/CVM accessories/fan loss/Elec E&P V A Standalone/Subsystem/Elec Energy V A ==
  volts_V : Inport
  curr_A : Inport  Port=2
  Gain : Gain  Gain=-1
  Integrator : Integrator  ZeroCross=off
  Integrator1 : Integrator  ZeroCross=off
  Integrator2 : Integrator  ZeroCross=off
  Mux : Mux  Inputs=2
  Neg : Fcn  Expr=u(1)*(u(1) <= 0)
  Pos : Fcn  Expr=u(1)*(u(1) >= 0)
  calc_Power_kW : Fcn  Expr=u(1)*u(2)/1000
  "total_kJ " : Outport
  "pos_kJ " : Outport  Port=2
  neg_kJ : Outport  Port=3
  pwr_kW : Outport  Port=4
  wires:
  curr_A/1 -> Mux/2
  volts_V/1 -> Mux/1
  Mux/1 -> calc_Power_kW/1
  Integrator/1 -> "total_kJ "/1
  Pos/1 -> Integrator1/1
  Neg/1 -> Integrator2/1
  Integrator2/1 -> Gain/1
  Integrator1/1 -> "pos_kJ "/1
  Gain/1 -> neg_kJ/1
  calc_Power_kW/1 -> Integrator/1, pwr_kW/1, Neg/1, Pos/1

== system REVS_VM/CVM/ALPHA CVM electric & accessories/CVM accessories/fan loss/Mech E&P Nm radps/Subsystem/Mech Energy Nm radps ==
  trq_Nm : Inport
  spd_radps : Inport  Port=2
  Gain : Gain  Gain=-1
  Integrator : Integrator  ZeroCross=off
  Integrator1 : Integrator  ZeroCross=off
  Integrator2 : Integrator  ZeroCross=off
  Mux : Mux  Inputs=2
  Neg : Fcn  Expr=u(1)*(u(1) <= 0)
  Pos : Fcn  Expr=u(1)*(u(1) >= 0)
  calc_Power_kW : Fcn  Expr=u(1)*u(2)/1000
  "total_kJ " : Outport
  "pos_kJ " : Outport  Port=2
  neg_kJ : Outport  Port=3
  pwr_kW : Outport  Port=4
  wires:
  calc_Power_kW/1 -> Pos/1, Neg/1, pwr_kW/1, Integrator/1
  Gain/1 -> neg_kJ/1
  Integrator1/1 -> "pos_kJ "/1
  Integrator2/1 -> Gain/1
  Neg/1 -> Integrator2/1
  Pos/1 -> Integrator1/1
  spd_radps/1 -> Mux/2
  trq_Nm/1 -> Mux/1
  Mux/1 -> calc_Power_kW/1
  Integrator/1 -> "total_kJ "/1

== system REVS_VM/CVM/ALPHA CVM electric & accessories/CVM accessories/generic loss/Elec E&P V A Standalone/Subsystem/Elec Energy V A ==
  volts_V : Inport
  curr_A : Inport  Port=2
  Gain : Gain  Gain=-1
  Integrator : Integrator  ZeroCross=off
  Integrator1 : Integrator  ZeroCross=off
  Integrator2 : Integrator  ZeroCross=off
  Mux : Mux  Inputs=2
  Neg : Fcn  Expr=u(1)*(u(1) <= 0)
  Pos : Fcn  Expr=u(1)*(u(1) >= 0)
  calc_Power_kW : Fcn  Expr=u(1)*u(2)/1000
  "total_kJ " : Outport
  "pos_kJ " : Outport  Port=2
  neg_kJ : Outport  Port=3
  pwr_kW : Outport  Port=4
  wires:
  curr_A/1 -> Mux/2
  volts_V/1 -> Mux/1
  Mux/1 -> calc_Power_kW/1
  Integrator/1 -> "total_kJ "/1
  Pos/1 -> Integrator1/1
  Neg/1 -> Integrator2/1
  Integrator2/1 -> Gain/1
  Integrator1/1 -> "pos_kJ "/1
  Gain/1 -> neg_kJ/1
  calc_Power_kW/1 -> Integrator/1, pwr_kW/1, Neg/1, Pos/1

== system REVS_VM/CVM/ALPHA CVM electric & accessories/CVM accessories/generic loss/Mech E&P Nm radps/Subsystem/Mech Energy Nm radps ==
  trq_Nm : Inport
  spd_radps : Inport  Port=2
  Gain : Gain  Gain=-1
  Integrator : Integrator  ZeroCross=off
  Integrator1 : Integrator  ZeroCross=off
  Integrator2 : Integrator  ZeroCross=off
  Mux : Mux  Inputs=2
  Neg : Fcn  Expr=u(1)*(u(1) <= 0)
  Pos : Fcn  Expr=u(1)*(u(1) >= 0)
  calc_Power_kW : Fcn  Expr=u(1)*u(2)/1000
  "total_kJ " : Outport
  "pos_kJ " : Outport  Port=2
  neg_kJ : Outport  Port=3
  pwr_kW : Outport  Port=4
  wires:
  calc_Power_kW/1 -> Pos/1, Neg/1, pwr_kW/1, Integrator/1
  Gain/1 -> neg_kJ/1
  Integrator1/1 -> "pos_kJ "/1
  Integrator2/1 -> Gain/1
  Neg/1 -> Integrator2/1
  Pos/1 -> Integrator1/1
  spd_radps/1 -> Mux/2
  trq_Nm/1 -> Mux/1
  Mux/1 -> calc_Power_kW/1
  Integrator/1 -> "total_kJ "/1

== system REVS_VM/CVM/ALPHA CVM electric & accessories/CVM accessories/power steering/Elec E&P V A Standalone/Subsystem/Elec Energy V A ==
  volts_V : Inport
  curr_A : Inport  Port=2
  Gain : Gain  Gain=-1
  Integrator : Integrator  ZeroCross=off
  Integrator1 : Integrator  ZeroCross=off
  Integrator2 : Integrator  ZeroCross=off
  Mux : Mux  Inputs=2
  Neg : Fcn  Expr=u(1)*(u(1) <= 0)
  Pos : Fcn  Expr=u(1)*(u(1) >= 0)
  calc_Power_kW : Fcn  Expr=u(1)*u(2)/1000
  "total_kJ " : Outport
  "pos_kJ " : Outport  Port=2
  neg_kJ : Outport  Port=3
  pwr_kW : Outport  Port=4
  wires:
  curr_A/1 -> Mux/2
  volts_V/1 -> Mux/1
  Mux/1 -> calc_Power_kW/1
  Integrator/1 -> "total_kJ "/1
  Pos/1 -> Integrator1/1
  Neg/1 -> Integrator2/1
  Integrator2/1 -> Gain/1
  Integrator1/1 -> "pos_kJ "/1
  Gain/1 -> neg_kJ/1
  calc_Power_kW/1 -> Integrator/1, pwr_kW/1, Neg/1, Pos/1

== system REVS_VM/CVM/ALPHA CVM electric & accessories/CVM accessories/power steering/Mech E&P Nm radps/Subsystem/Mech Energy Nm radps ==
  trq_Nm : Inport
  spd_radps : Inport  Port=2
  Gain : Gain  Gain=-1
  Integrator : Integrator  ZeroCross=off
  Integrator1 : Integrator  ZeroCross=off
  Integrator2 : Integrator  ZeroCross=off
  Mux : Mux  Inputs=2
  Neg : Fcn  Expr=u(1)*(u(1) <= 0)
  Pos : Fcn  Expr=u(1)*(u(1) >= 0)
  calc_Power_kW : Fcn  Expr=u(1)*u(2)/1000
  "total_kJ " : Outport
  "pos_kJ " : Outport  Port=2
  neg_kJ : Outport  Port=3
  pwr_kW : Outport  Port=4
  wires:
  calc_Power_kW/1 -> Pos/1, Neg/1, pwr_kW/1, Integrator/1
  Gain/1 -> neg_kJ/1
  Integrator1/1 -> "pos_kJ "/1
  Integrator2/1 -> Gain/1
  Neg/1 -> Integrator2/1
  Pos/1 -> Integrator1/1
  spd_radps/1 -> Mux/2
  trq_Nm/1 -> Mux/1
  Mux/1 -> calc_Power_kW/1
  Integrator/1 -> "total_kJ "/1

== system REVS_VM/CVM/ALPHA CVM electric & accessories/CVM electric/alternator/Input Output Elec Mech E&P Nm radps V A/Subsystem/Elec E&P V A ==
  volts_V : Inport
  curr_A : Inport  Port=2
  Compare To Constant : simulink/Logic and Bit Operations/Compare To Constant  relop=>=  const=1  OutDataTypeStr=boolean
  Constant : Constant  Value=VerboseSignal
  Subsystem : Subsystem
  pos_kJ : Outport
  neg_kJ : Outport  Port=2
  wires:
  volts_V/1 -> Subsystem/1(volts_V)
  curr_A/1 -> Subsystem/2(curr_A)
  Subsystem/1(pos_kJ) -> pos_kJ/1
  Subsystem/2(neg_kJ) -> neg_kJ/1
  Compare To Constant/1 -> Subsystem/Enable
  Constant/1 -> Compare To Constant/1

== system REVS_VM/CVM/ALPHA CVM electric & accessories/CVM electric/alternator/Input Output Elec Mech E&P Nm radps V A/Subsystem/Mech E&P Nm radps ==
  " trq_Nm" : Inport
  spd_radps : Inport  Port=2
  iner_kgm2 : Inport  Port=3
  Compare To Constant : simulink/Logic and Bit Operations/Compare To Constant  relop=>=  const=1  OutDataTypeStr=boolean
  Constant : Constant  Value=VerboseSignal
  Subsystem : Subsystem
  pos_kJ : Outport
  neg_kJ : Outport  Port=2
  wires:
  " trq_Nm"/1 -> Subsystem/1(" trq_Nm")
  spd_radps/1 -> Subsystem/2(spd_radps)
  iner_kgm2/1 -> Subsystem/3(iner_kgm2)
  Compare To Constant/1 -> Subsystem/Enable
  Subsystem/1(pos_kJ) -> pos_kJ/1
  Subsystem/2(neg_kJ) -> neg_kJ/1
  Constant/1 -> Compare To Constant/1

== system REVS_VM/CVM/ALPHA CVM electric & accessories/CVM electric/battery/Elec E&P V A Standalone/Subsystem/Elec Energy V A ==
  volts_V : Inport
  curr_A : Inport  Port=2
  Gain : Gain  Gain=-1
  Integrator : Integrator  ZeroCross=off
  Integrator1 : Integrator  ZeroCross=off
  Integrator2 : Integrator  ZeroCross=off
  Mux : Mux  Inputs=2
  Neg : Fcn  Expr=u(1)*(u(1) <= 0)
  Pos : Fcn  Expr=u(1)*(u(1) >= 0)
  calc_Power_kW : Fcn  Expr=u(1)*u(2)/1000
  "total_kJ " : Outport
  "pos_kJ " : Outport  Port=2
  neg_kJ : Outport  Port=3
  pwr_kW : Outport  Port=4
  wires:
  curr_A/1 -> Mux/2
  volts_V/1 -> Mux/1
  Mux/1 -> calc_Power_kW/1
  Integrator/1 -> "total_kJ "/1
  Pos/1 -> Integrator1/1
  Neg/1 -> Integrator2/1
  Integrator2/1 -> Gain/1
  Integrator1/1 -> "pos_kJ "/1
  Gain/1 -> neg_kJ/1
  calc_Power_kW/1 -> Integrator/1, pwr_kW/1, Neg/1, Pos/1

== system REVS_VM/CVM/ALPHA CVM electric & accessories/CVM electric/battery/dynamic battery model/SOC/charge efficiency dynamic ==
  bus : Inport
  Bus Selector : BusSelector  OutputSignals=gb.gb_cmd_gear,gb_spd_in_radps,ctrl.gb_line_press_bar
  Lookup : Lookup_n-D  NumberOfTableDimensions=10  BreakpointsForDimension1=LookupStructure.axis_1.breakpoints  BreakpointsForDimension2=LookupStructure.axis_2.breakpoints  BreakpointsForDimension3=LookupStructure.axis_3.breakpoints  BreakpointsForDimension4=LookupStructure.axis_4.breakpoints  BreakpointsForDimension5=LookupStructure.axis_5.breakpoints  BreakpointsForDimension6=LookupStructure.axis_6.breakpoints  BreakpointsForDimension7=LookupStructure.axis_7.breakpoints  BreakpointsForDimension8=LookupStructure.axis_8.breakpoints  BreakpointsForDimension9=LookupStructure.axis_9.breakpoints  BreakpointsForDimension10=LookupStructure.axis_10.breakpoints  IndexSearchMethod=Linear search  BeginIndexSearchUsingPreviousIndexResult=on  Table=LookupStructure.table  InternalRulePriority=Speed  RndMeth=Simplest  SupportTunableTableSize=on  MaximumIndicesForEachDimension=LookupStructure.table_size
  out : Outport
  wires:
  bus/1 -> Bus Selector/1
  Lookup/1 -> out/1

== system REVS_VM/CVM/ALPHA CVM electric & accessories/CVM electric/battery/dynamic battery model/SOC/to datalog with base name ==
  Var : Inport
  Constant : Constant  Value=VerboseSignal
  Constant1 : Constant  Value=VerboseLevel
  Relational Operator : RelationalOperator  OutDataTypeStr=boolean  ZeroCross=off
  Subsystem : Subsystem
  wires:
  Constant1/1 -> Relational Operator/2
  Relational Operator/1 -> Subsystem/Enable
  Constant/1 -> Relational Operator/1
  Var/1 -> Subsystem/1(Var)

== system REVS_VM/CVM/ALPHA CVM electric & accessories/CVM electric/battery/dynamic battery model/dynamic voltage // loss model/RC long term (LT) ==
  bus_in : Inport
  Add2 : Sum  Inputs=+-
  Bus Selector : BusSelector  OutputSignals=pack_curr_A
  Cp long term : Subsystem
  Integrator : Integrator
  Product4 : Product  Inputs=*/
  Product5 : Product  Inputs=*/
  Rp long term : Subsystem
  to datalog with base name : Subsystem
  to datalog with base name1 : Subsystem
  to datalog with base name2 : Subsystem
  use 2nd order : Gain  Gain=battery.use_second_order_model
  RC_LT_V : Outport
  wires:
  use 2nd order/1 -> RC_LT_V/1, to datalog with base name/1(Var)
  Cp long term/1(Cp_LT_Farad) -> to datalog with base name2/1(Var), Product4/2
  Add2/1 -> Product4/1
  Product5/1 -> Add2/2  "I LT"
  Product4/1 -> Integrator/1
  Integrator/1 -> use 2nd order/1, Product5/1
  Bus Selector/1 -> Add2/1  "<pack_curr_A>"
  Rp long term/1(Rp_LT_Ohm) -> to datalog with base name1/1(Var), Product5/2
  bus_in/1 -> Rp long term/1(bus_in), Cp long term/1(bus_in), Bus Selector/1
